(* Logix 5000 AddOnInstructionDefinition export HI1734_Faceplate_IT_AOI; software revision 30.00; part 2 of 2 *)
(* tags used below, declared in another part *)
   Inp_hi1734 : HI:1734_WS:I:0;
   Out_hi1734 : HI:1734_WS:O:0;
   IT_Status : DINT;   // Integrated Technician status indication
   pm_49C8 : REAL;   // WAVERSAVER VAR ref 1
   pm_49C4 : REAL;   // WAVERSAVER VAR ch 4
   pm_49C5 : REAL;   // WAVERSAVER VAR ch 5
   pm_49C6 : REAL;   // WAVERSAVER VAR ch 6
   pm_49C7 : REAL;   // WAVERSAVER VAR ch 7
   pm_49C9 : REAL;   // WAVERSAVER VAR ref 2
   pm_49D0 : DINT;   // RAW VAR results ch 0
   pm_49D1 : DINT;   // RAW VAR results ch 1
   pm_49D2 : DINT;   // RAW VAR results ch 2
   pm_49D3 : DINT;   // RAW VAR results ch 3
   pm_49D8 : DINT;   // RAW VAR results ref 1
   pm_49D4 : DINT;   // RAW VAR results ch 4
   pm_49D5 : DINT;   // RAW VAR results ch 5
   pm_49D6 : DINT;   // RAW VAR results ch 6
   pm_49D7 : DINT;   // RAW VAR results ch 7
   pm_49D9 : DINT;   // RAW VAR results ref 2
   pm_49E0 : DINT;   // WAVERSAVER VAR results ch 0
   pm_49E1 : DINT;   // WAVERSAVER VAR results ch 1
   pm_49E2 : DINT;   // WAVERSAVER VAR results ch 2
   pm_49E3 : DINT;   // WAVERSAVER VAR results ch 3
   pm_49E8 : DINT;   // WAVERSAVER VAR results ref 1
   pm_49E4 : DINT;   // WAVERSAVER VAR results ch 4
   pm_49E5 : DINT;   // WAVERSAVER VAR results ch 5
   pm_49E6 : DINT;   // WAVERSAVER VAR results ch 6
   pm_49E7 : DINT;   // WAVERSAVER VAR results ch 7
   pm_49E9 : DINT;   // WAVERSAVER VAR results ref 2
   rd_rtz : INT;   // return to zero status
   pm_49F0 : DINT;   // RTZ ch 0
   pm_49F1 : DINT;   // RTZ ch 1
   pm_49F2 : DINT;   // RTZ ch 2
   pm_49F3 : DINT;   // RTZ ch 3
   pm_49F4 : DINT;   // RTZ ch 4
   pm_49F5 : DINT;   // RTZ ch 5
   pm_49F6 : DINT;   // RTZ ch 6
   pm_49F7 : DINT;   // RTZ ch 7
   pm_498C : DINT;   // RTZ combined
   IT_running_status : DINT;   // running/status indication
   rd_ws_var : INT;   // trigger to read WAVERSAVER variation
   rd_raw_rst : INT;   // trigger to read raw variation results
   rd_ws_rst : INT;   // trigger to read WAVERSAVER results
   start_timer116 : BOOL;   // process control bit
   delay116 : TIMER;   // delay to allow process to complete
   start_timer117 : BOOL;   // process control bit
   delay117 : TIMER;   // delay to allow process to complete
   start_timer118 : BOOL;   // process control bit
   start_timer119 : BOOL;   // process control bit
   delay118 : TIMER;   // delay to allow process to complete
   delay119 : TIMER;   // delay to allow process to complete
   start_timer120 : BOOL;   // process control bit
   delay120 : TIMER;   // delay to allow process to complete
   start_timer121 : BOOL;   // process control bit
   delay121 : TIMER;   // delay to allow process to complete
   start_timer122 : BOOL;   // process control bit
   delay122 : TIMER;   // delay to allow process to complete
   start_timer123 : BOOL;   // process control bit
   delay123 : TIMER;   // delay to allow process to complete
   start_timer124 : BOOL;   // process control bit
   delay124 : TIMER;   // delay to allow process to complete
   start_timer125 : BOOL;   // process control bit
   delay125 : TIMER;   // delay to allow process to complete
   start_timer126 : BOOL;   // process control bit
   delay126 : TIMER;   // delay to allow process to complete
   start_timer127 : BOOL;   // process control bit
   delay127 : TIMER;   // delay to allow process to complete
   start_timer128 : BOOL;   // process control bit
   delay128 : TIMER;   // delay to allow process to complete
   start_timer129 : BOOL;   // process control bit
   delay129 : TIMER;   // delay to allow process to complete
   start_timer130 : BOOL;   // process control bit
   delay130 : TIMER;   // delay to allow process to complete
   start_timer131 : BOOL;   // process control bit
   delay131 : TIMER;   // delay to allow process to complete
   start_timer132 : BOOL;   // process control bit
   delay132 : TIMER;   // delay to allow process to complete
   start_timer133 : BOOL;   // process control bit
   delay133 : TIMER;   // delay to allow process to complete
   clear_status : BOOL;   // process control bit
   delay138 : TIMER;   // delay to allow process to complete
   rd_jbox_2_too : BOOL;   // Process control bit
(* HI1734_Faceplate_IT_AOI, continued *)

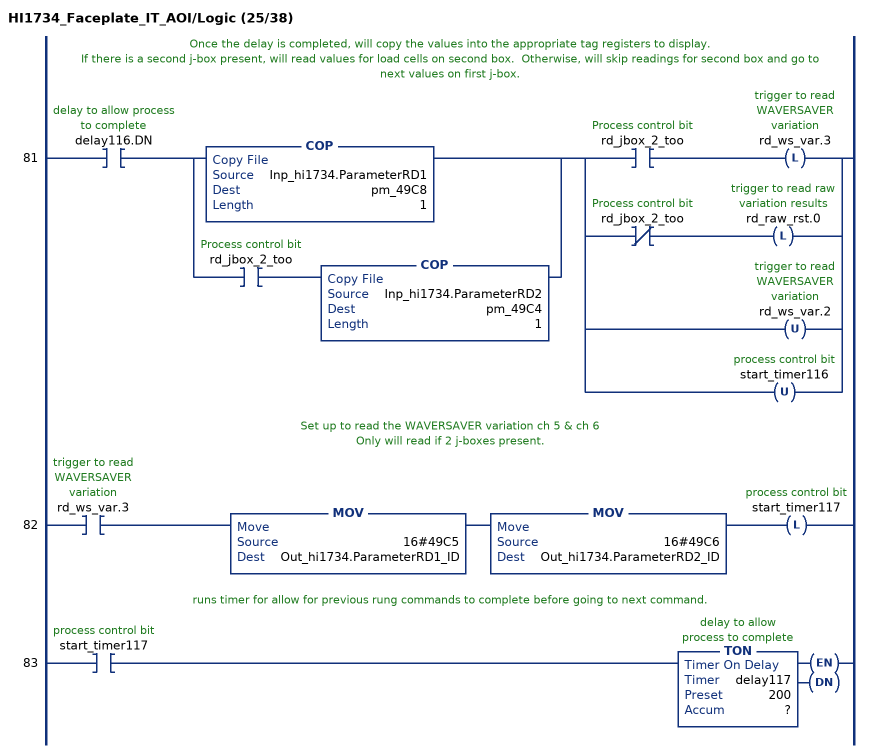
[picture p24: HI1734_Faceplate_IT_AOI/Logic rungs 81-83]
   // Once the delay is completed, will copy the values into the appropriate tag registers to display.
   // If there is a second j-box present, will read values for load cells on second box.  Otherwise, will skip readings for second box and go to next values on first j-box.
   81: XIC(delay116.DN)[COP(Inp_hi1734.ParameterRD1,pm_49C8,1) ,XIC(rd_jbox_2_too) COP(Inp_hi1734.ParameterRD2,pm_49C4,1) ][XIC(rd_jbox_2_too) OTL(rd_ws_var.3) ,XIO(rd_jbox_2_too) OTL(rd_raw_rst.0) ,OTU(rd_ws_var.2) ,OTU(start_timer116) ];
   // Set up to read the WAVERSAVER variation ch 5 & ch 6
   // Only will read if 2 j-boxes present.
   82: XIC(rd_ws_var.3)MOV(16#49C5,Out_hi1734.ParameterRD1_ID)MOV(16#49C6,Out_hi1734.ParameterRD2_ID)OTL(start_timer117);
   // runs timer for allow for previous rung commands to complete before going to next command.
   83: XIC(start_timer117)TON(delay117,?,?);
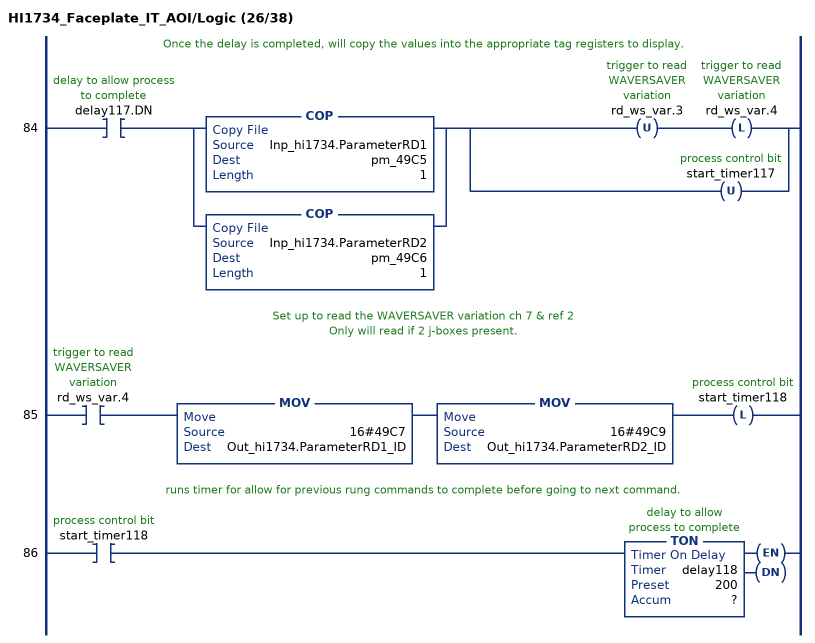
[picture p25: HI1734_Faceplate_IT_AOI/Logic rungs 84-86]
   // Once the delay is completed, will copy the values into the appropriate tag registers to display.
   84: XIC(delay117.DN)[COP(Inp_hi1734.ParameterRD1,pm_49C5,1) ,COP(Inp_hi1734.ParameterRD2,pm_49C6,1) ][OTU(rd_ws_var.3) OTL(rd_ws_var.4) ,OTU(start_timer117) ];
   // Set up to read the WAVERSAVER variation ch 7 & ref 2
   // Only will read if 2 j-boxes present.
   85: XIC(rd_ws_var.4)MOV(16#49C7,Out_hi1734.ParameterRD1_ID)MOV(16#49C9,Out_hi1734.ParameterRD2_ID)OTL(start_timer118);
   // runs timer for allow for previous rung commands to complete before going to next command.
   86: XIC(start_timer118)TON(delay118,?,?);
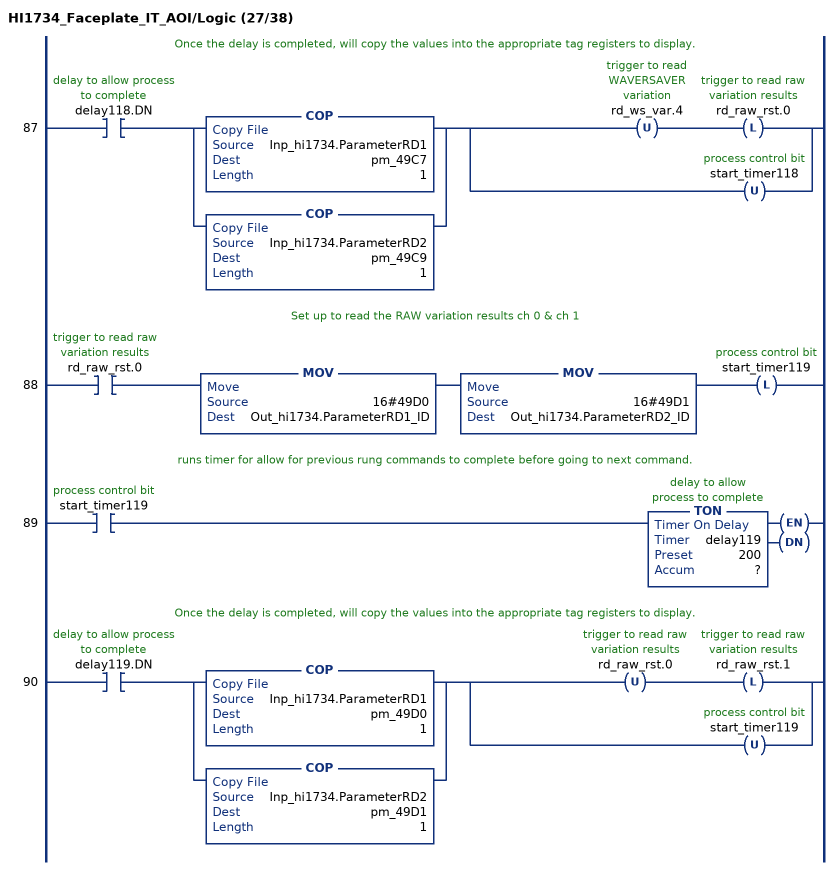
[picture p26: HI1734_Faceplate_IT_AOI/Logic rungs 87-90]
   // Once the delay is completed, will copy the values into the appropriate tag registers to display.
   87: XIC(delay118.DN)[COP(Inp_hi1734.ParameterRD1,pm_49C7,1) ,COP(Inp_hi1734.ParameterRD2,pm_49C9,1) ][OTU(rd_ws_var.4) OTL(rd_raw_rst.0) ,OTU(start_timer118) ];
   // Set up to read the RAW variation results ch 0 & ch 1
   88: XIC(rd_raw_rst.0)MOV(16#49D0,Out_hi1734.ParameterRD1_ID)MOV(16#49D1,Out_hi1734.ParameterRD2_ID)OTL(start_timer119);
   // runs timer for allow for previous rung commands to complete before going to next command.
   89: XIC(start_timer119)TON(delay119,?,?);
   // Once the delay is completed, will copy the values into the appropriate tag registers to display.
   90: XIC(delay119.DN)[COP(Inp_hi1734.ParameterRD1,pm_49D0,1) ,COP(Inp_hi1734.ParameterRD2,pm_49D1,1) ][OTU(rd_raw_rst.0) OTL(rd_raw_rst.1) ,OTU(start_timer119) ];
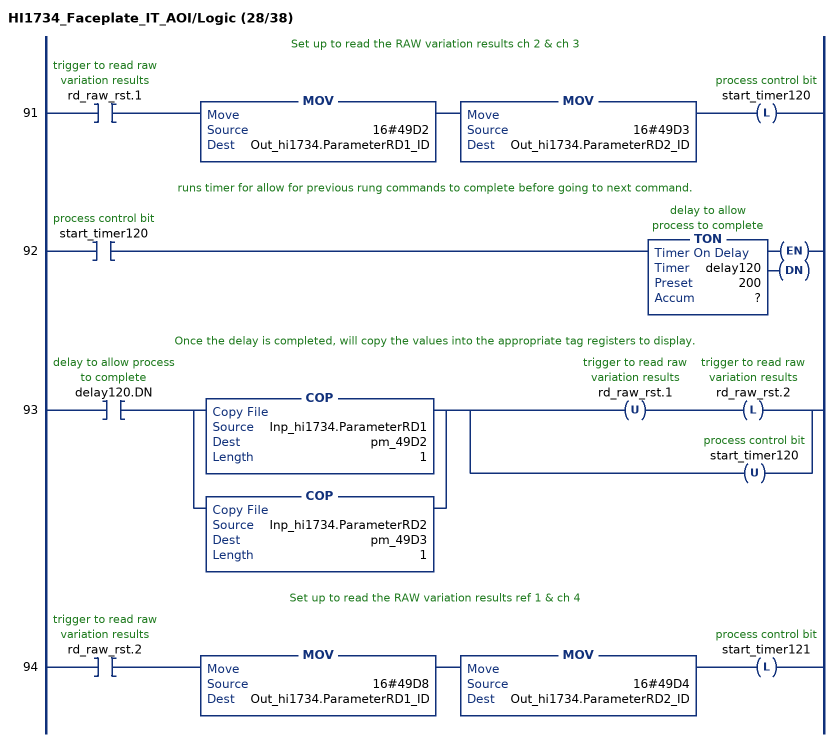
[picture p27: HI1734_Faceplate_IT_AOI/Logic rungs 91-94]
   // Set up to read the RAW variation results ch 2 & ch 3
   91: XIC(rd_raw_rst.1)MOV(16#49D2,Out_hi1734.ParameterRD1_ID)MOV(16#49D3,Out_hi1734.ParameterRD2_ID)OTL(start_timer120);
   // runs timer for allow for previous rung commands to complete before going to next command.
   92: XIC(start_timer120)TON(delay120,?,?);
   // Once the delay is completed, will copy the values into the appropriate tag registers to display.
   93: XIC(delay120.DN)[COP(Inp_hi1734.ParameterRD1,pm_49D2,1) ,COP(Inp_hi1734.ParameterRD2,pm_49D3,1) ][OTU(rd_raw_rst.1) OTL(rd_raw_rst.2) ,OTU(start_timer120) ];
   // Set up to read the RAW variation results ref 1 & ch 4
   94: XIC(rd_raw_rst.2)MOV(16#49D8,Out_hi1734.ParameterRD1_ID)MOV(16#49D4,Out_hi1734.ParameterRD2_ID)OTL(start_timer121);
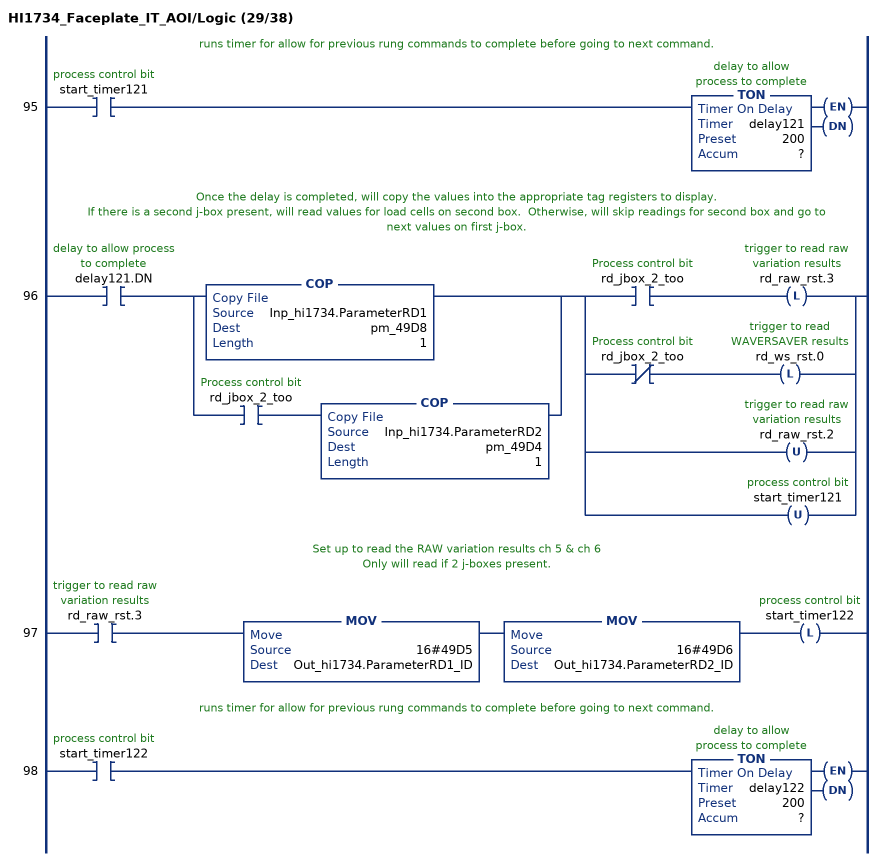
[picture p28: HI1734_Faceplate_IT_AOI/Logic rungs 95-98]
   // runs timer for allow for previous rung commands to complete before going to next command.
   95: XIC(start_timer121)TON(delay121,?,?);
   // Once the delay is completed, will copy the values into the appropriate tag registers to display.
   // If there is a second j-box present, will read values for load cells on second box.  Otherwise, will skip readings for second box and go to next values on first j-box.
   96: XIC(delay121.DN)[COP(Inp_hi1734.ParameterRD1,pm_49D8,1) ,XIC(rd_jbox_2_too) COP(Inp_hi1734.ParameterRD2,pm_49D4,1) ][XIC(rd_jbox_2_too) OTL(rd_raw_rst.3) ,XIO(rd_jbox_2_too) OTL(rd_ws_rst.0) ,OTU(rd_raw_rst.2) ,OTU(start_timer121) ];
   // Set up to read the RAW variation results ch 5 & ch 6
   // Only will read if 2 j-boxes present.
   97: XIC(rd_raw_rst.3)MOV(16#49D5,Out_hi1734.ParameterRD1_ID)MOV(16#49D6,Out_hi1734.ParameterRD2_ID)OTL(start_timer122);
   // runs timer for allow for previous rung commands to complete before going to next command.
   98: XIC(start_timer122)TON(delay122,?,?);
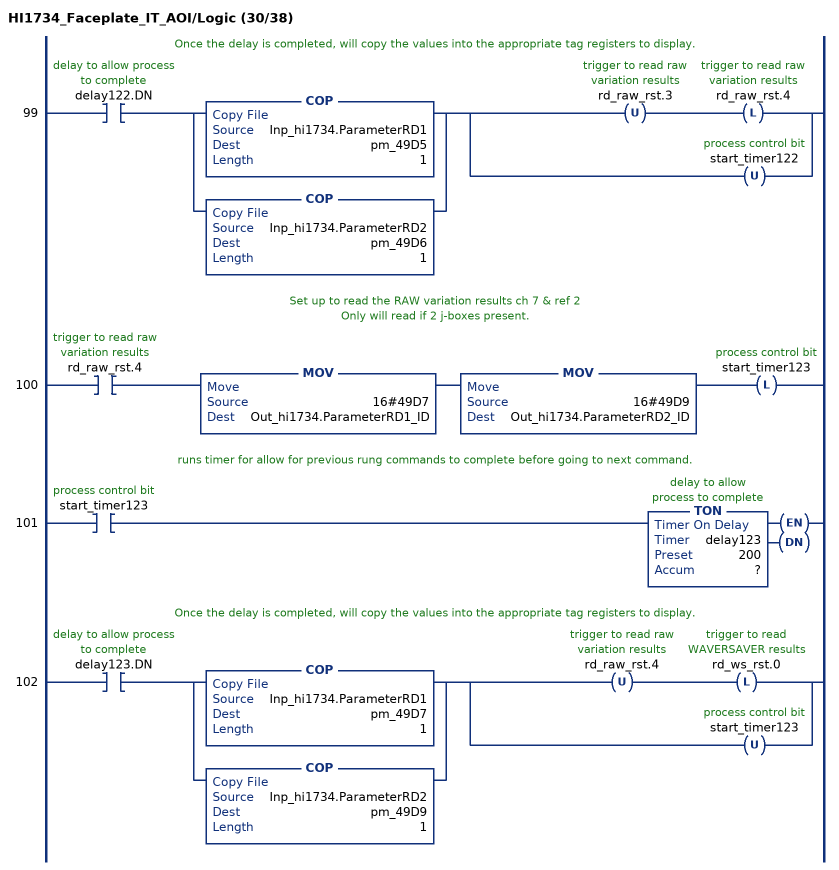
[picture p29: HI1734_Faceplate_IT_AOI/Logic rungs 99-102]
   // Once the delay is completed, will copy the values into the appropriate tag registers to display.
   99: XIC(delay122.DN)[COP(Inp_hi1734.ParameterRD1,pm_49D5,1) ,COP(Inp_hi1734.ParameterRD2,pm_49D6,1) ][OTU(rd_raw_rst.3) OTL(rd_raw_rst.4) ,OTU(start_timer122) ];
   // Set up to read the RAW variation results ch 7 & ref 2
   // Only will read if 2 j-boxes present.
   100: XIC(rd_raw_rst.4)MOV(16#49D7,Out_hi1734.ParameterRD1_ID)MOV(16#49D9,Out_hi1734.ParameterRD2_ID)OTL(start_timer123);
   // runs timer for allow for previous rung commands to complete before going to next command.
   101: XIC(start_timer123)TON(delay123,?,?);
   // Once the delay is completed, will copy the values into the appropriate tag registers to display.
   102: XIC(delay123.DN)[COP(Inp_hi1734.ParameterRD1,pm_49D7,1) ,COP(Inp_hi1734.ParameterRD2,pm_49D9,1) ][OTU(rd_raw_rst.4) OTL(rd_ws_rst.0) ,OTU(start_timer123) ];
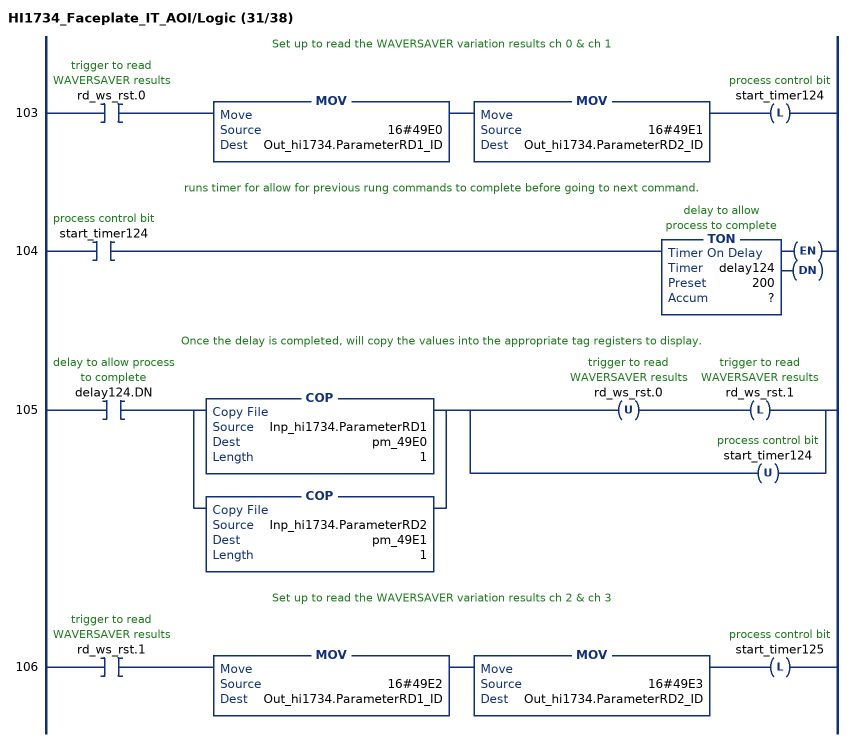
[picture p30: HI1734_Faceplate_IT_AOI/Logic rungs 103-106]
   // Set up to read the WAVERSAVER variation results ch 0 & ch 1
   103: XIC(rd_ws_rst.0)MOV(16#49E0,Out_hi1734.ParameterRD1_ID)MOV(16#49E1,Out_hi1734.ParameterRD2_ID)OTL(start_timer124);
   // runs timer for allow for previous rung commands to complete before going to next command.
   104: XIC(start_timer124)TON(delay124,?,?);
   // Once the delay is completed, will copy the values into the appropriate tag registers to display.
   105: XIC(delay124.DN)[COP(Inp_hi1734.ParameterRD1,pm_49E0,1) ,COP(Inp_hi1734.ParameterRD2,pm_49E1,1) ][OTU(rd_ws_rst.0) OTL(rd_ws_rst.1) ,OTU(start_timer124) ];
   // Set up to read the WAVERSAVER variation results ch 2 & ch 3
   106: XIC(rd_ws_rst.1)MOV(16#49E2,Out_hi1734.ParameterRD1_ID)MOV(16#49E3,Out_hi1734.ParameterRD2_ID)OTL(start_timer125);
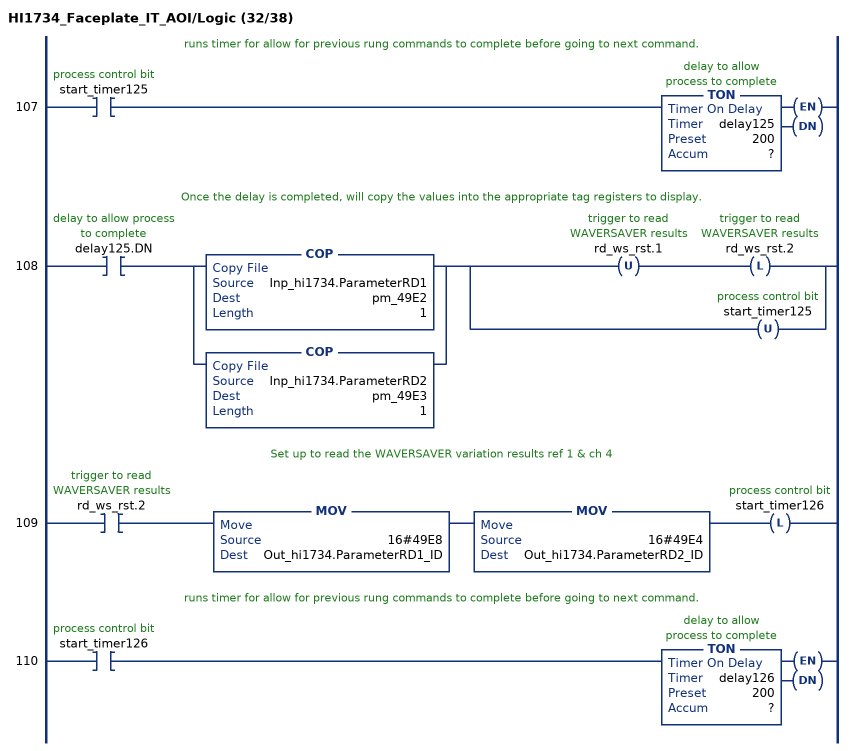
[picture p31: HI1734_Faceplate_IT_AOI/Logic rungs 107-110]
   // runs timer for allow for previous rung commands to complete before going to next command.
   107: XIC(start_timer125)TON(delay125,?,?);
   // Once the delay is completed, will copy the values into the appropriate tag registers to display.
   108: XIC(delay125.DN)[COP(Inp_hi1734.ParameterRD1,pm_49E2,1) ,COP(Inp_hi1734.ParameterRD2,pm_49E3,1) ][OTU(rd_ws_rst.1) OTL(rd_ws_rst.2) ,OTU(start_timer125) ];
   // Set up to read the WAVERSAVER variation results ref 1 & ch 4
   109: XIC(rd_ws_rst.2)MOV(16#49E8,Out_hi1734.ParameterRD1_ID)MOV(16#49E4,Out_hi1734.ParameterRD2_ID)OTL(start_timer126);
   // runs timer for allow for previous rung commands to complete before going to next command.
   110: XIC(start_timer126)TON(delay126,?,?);
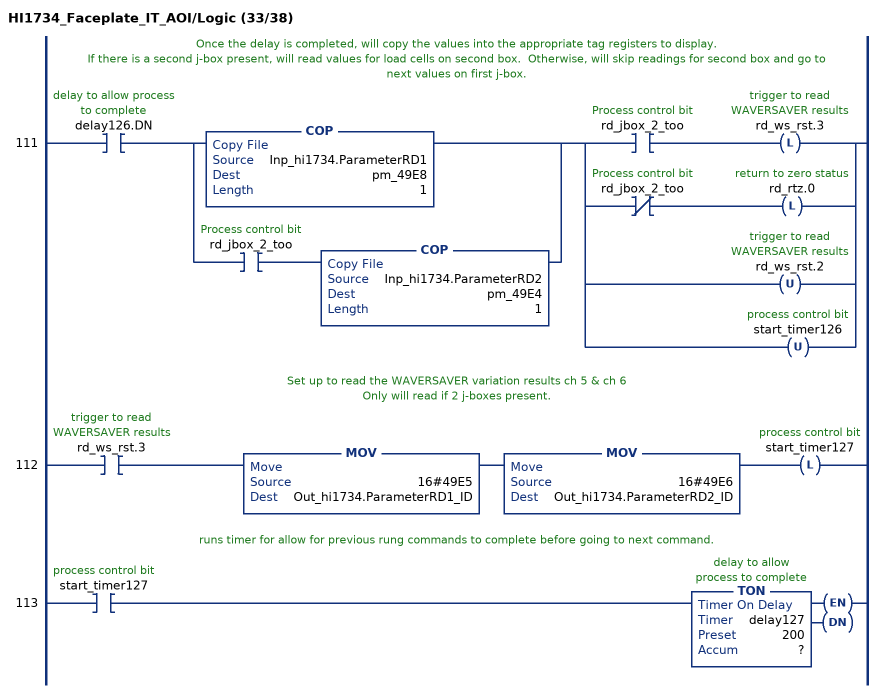
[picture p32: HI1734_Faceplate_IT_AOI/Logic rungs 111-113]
   // Once the delay is completed, will copy the values into the appropriate tag registers to display.
   // If there is a second j-box present, will read values for load cells on second box.  Otherwise, will skip readings for second box and go to next values on first j-box.
   111: XIC(delay126.DN)[COP(Inp_hi1734.ParameterRD1,pm_49E8,1) ,XIC(rd_jbox_2_too) COP(Inp_hi1734.ParameterRD2,pm_49E4,1) ][XIC(rd_jbox_2_too) OTL(rd_ws_rst.3) ,XIO(rd_jbox_2_too) OTL(rd_rtz.0) ,OTU(rd_ws_rst.2) ,OTU(start_timer126) ];
   // Set up to read the WAVERSAVER variation results ch 5 & ch 6
   // Only will read if 2 j-boxes present.
   112: XIC(rd_ws_rst.3)MOV(16#49E5,Out_hi1734.ParameterRD1_ID)MOV(16#49E6,Out_hi1734.ParameterRD2_ID)OTL(start_timer127);
   // runs timer for allow for previous rung commands to complete before going to next command.
   113: XIC(start_timer127)TON(delay127,?,?);
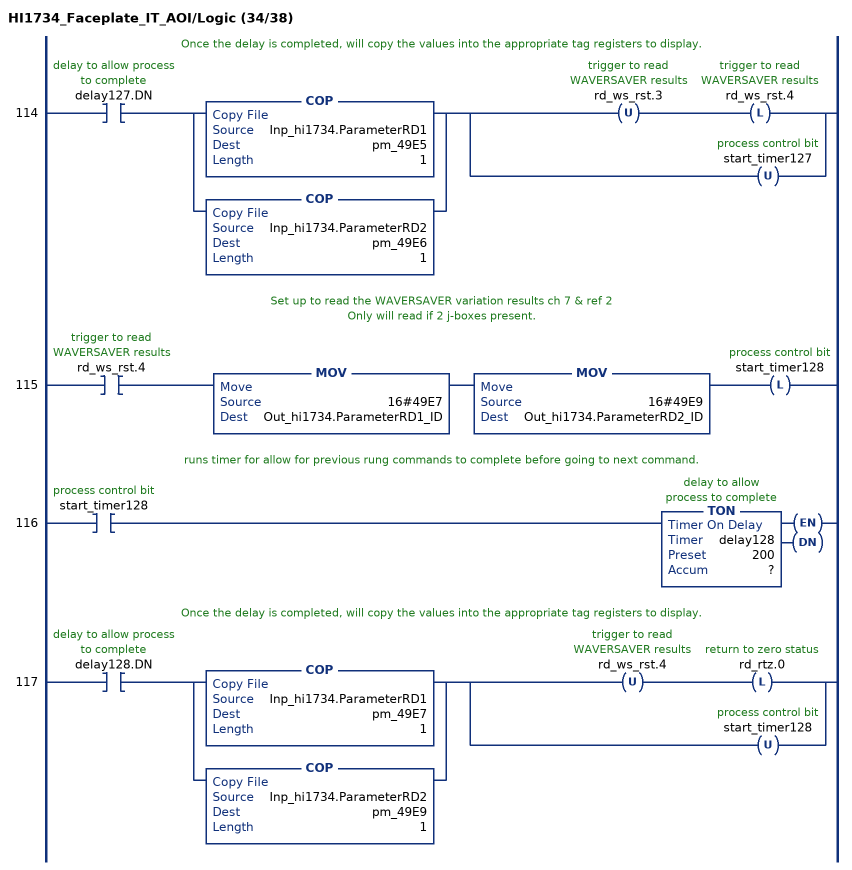
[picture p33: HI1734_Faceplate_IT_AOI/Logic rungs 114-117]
   // Once the delay is completed, will copy the values into the appropriate tag registers to display.
   114: XIC(delay127.DN)[COP(Inp_hi1734.ParameterRD1,pm_49E5,1) ,COP(Inp_hi1734.ParameterRD2,pm_49E6,1) ][OTU(rd_ws_rst.3) OTL(rd_ws_rst.4) ,OTU(start_timer127) ];
   // Set up to read the WAVERSAVER variation results ch 7 & ref 2
   //  Only will read if 2 j-boxes present.
   115: XIC(rd_ws_rst.4)MOV(16#49E7,Out_hi1734.ParameterRD1_ID)MOV(16#49E9,Out_hi1734.ParameterRD2_ID)OTL(start_timer128);
   // runs timer for allow for previous rung commands to complete before going to next command.
   116: XIC(start_timer128)TON(delay128,?,?);
   // Once the delay is completed, will copy the values into the appropriate tag registers to display.
   117: XIC(delay128.DN)[COP(Inp_hi1734.ParameterRD1,pm_49E7,1) ,COP(Inp_hi1734.ParameterRD2,pm_49E9,1) ][OTU(rd_ws_rst.4) OTL(rd_rtz.0) ,OTU(start_timer128) ];
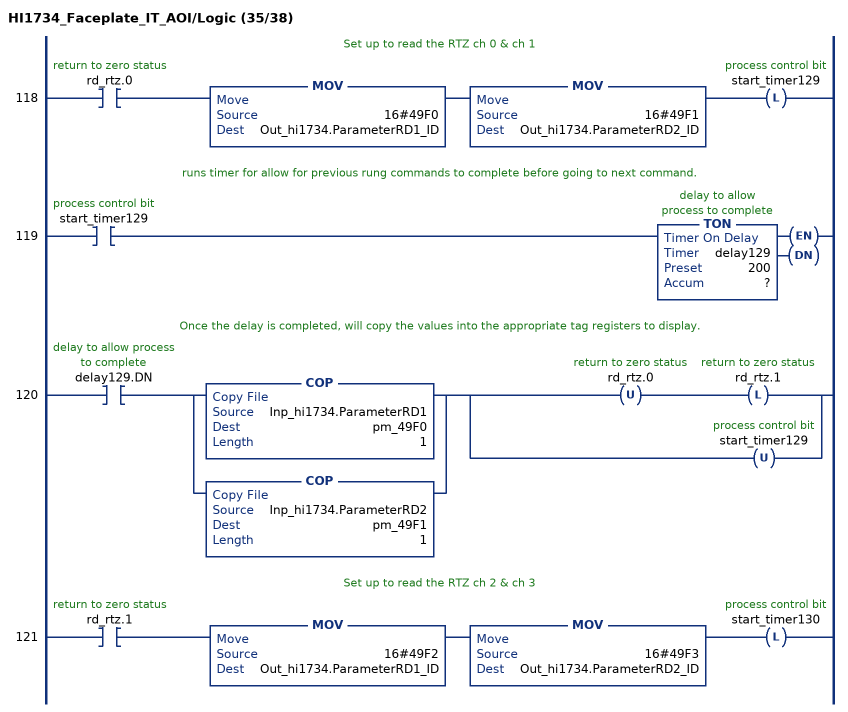
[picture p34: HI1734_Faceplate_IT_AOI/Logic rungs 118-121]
   // Set up to read the RTZ ch 0 & ch 1
   118: XIC(rd_rtz.0)MOV(16#49F0,Out_hi1734.ParameterRD1_ID)MOV(16#49F1,Out_hi1734.ParameterRD2_ID)OTL(start_timer129);
   // runs timer for allow for previous rung commands to complete before going to next command.
   119: XIC(start_timer129)TON(delay129,?,?);
   // Once the delay is completed, will copy the values into the appropriate tag registers to display.
   120: XIC(delay129.DN)[COP(Inp_hi1734.ParameterRD1,pm_49F0,1) ,COP(Inp_hi1734.ParameterRD2,pm_49F1,1) ][OTU(rd_rtz.0) OTL(rd_rtz.1) ,OTU(start_timer129) ];
   // Set up to read the RTZ ch 2 & ch 3
   121: XIC(rd_rtz.1)MOV(16#49F2,Out_hi1734.ParameterRD1_ID)MOV(16#49F3,Out_hi1734.ParameterRD2_ID)OTL(start_timer130);
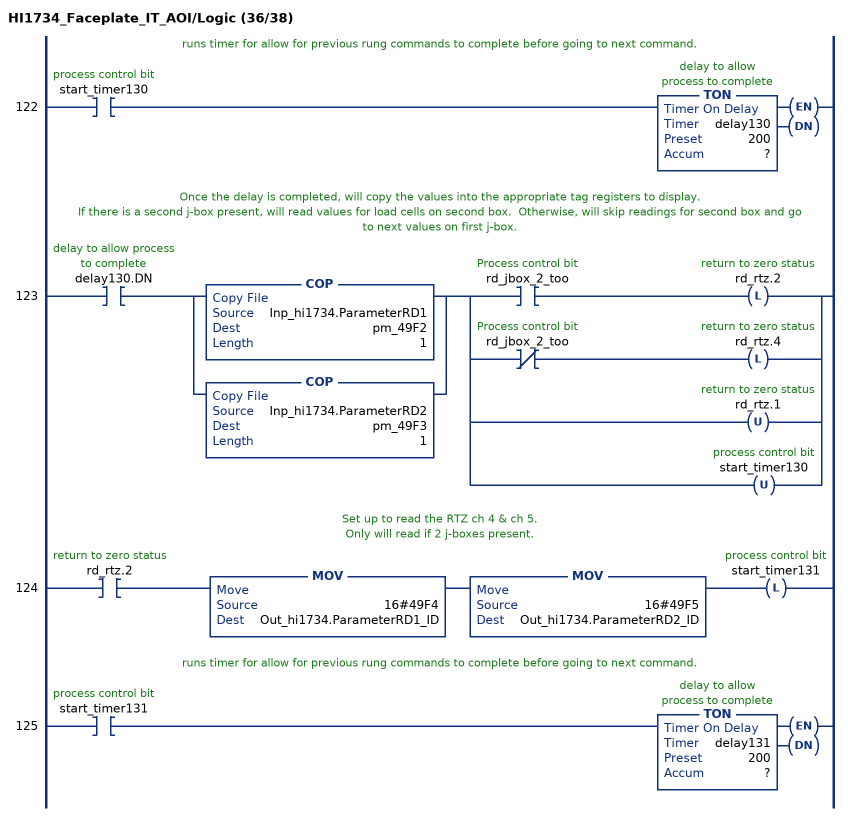
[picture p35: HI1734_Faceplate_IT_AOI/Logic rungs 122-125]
   // runs timer for allow for previous rung commands to complete before going to next command.
   122: XIC(start_timer130)TON(delay130,?,?);
   // Once the delay is completed, will copy the values into the appropriate tag registers to display.
   // If there is a second j-box present, will read values for load cells on second box.  Otherwise, will skip readings for second box and go to next values on first j-box.
   123: XIC(delay130.DN)[COP(Inp_hi1734.ParameterRD1,pm_49F2,1) ,COP(Inp_hi1734.ParameterRD2,pm_49F3,1) ][XIC(rd_jbox_2_too) OTL(rd_rtz.2) ,XIO(rd_jbox_2_too) OTL(rd_rtz.4) ,OTU(rd_rtz.1) ,OTU(start_timer130) ];
   // Set up to read the RTZ ch 4 & ch 5.
   // Only will read if 2 j-boxes present.
   124: XIC(rd_rtz.2)MOV(16#49F4,Out_hi1734.ParameterRD1_ID)MOV(16#49F5,Out_hi1734.ParameterRD2_ID)OTL(start_timer131);
   // runs timer for allow for previous rung commands to complete before going to next command.
   125: XIC(start_timer131)TON(delay131,?,?);
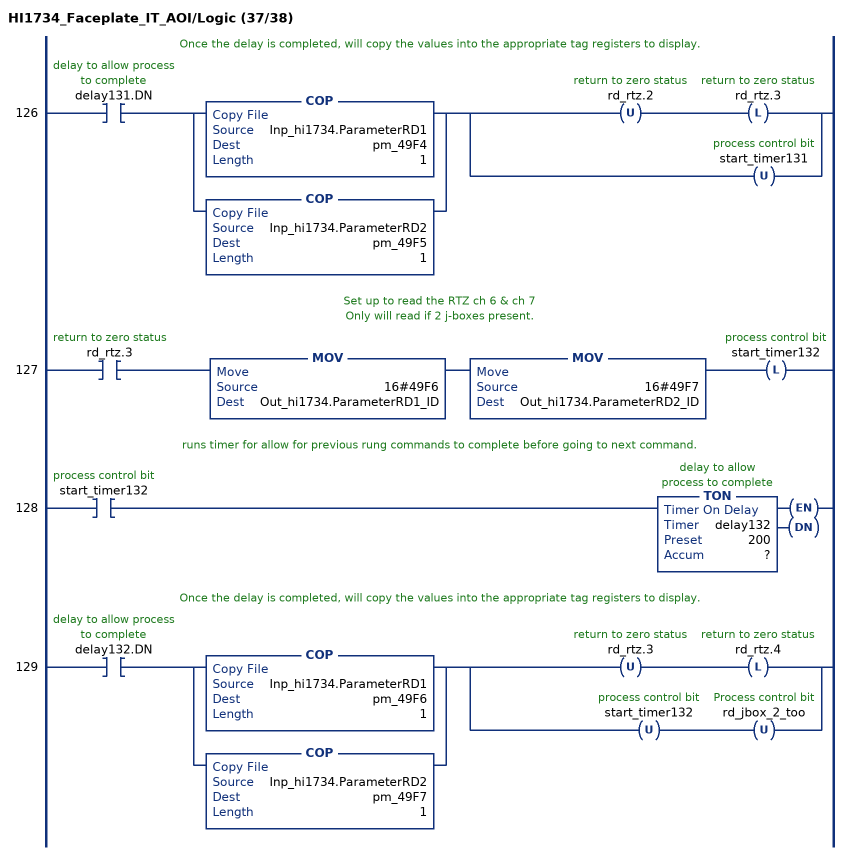
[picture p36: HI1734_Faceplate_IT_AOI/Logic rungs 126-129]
   // Once the delay is completed, will copy the values into the appropriate tag registers to display.
   126: XIC(delay131.DN)[COP(Inp_hi1734.ParameterRD1,pm_49F4,1) ,COP(Inp_hi1734.ParameterRD2,pm_49F5,1) ][OTU(rd_rtz.2) OTL(rd_rtz.3) ,OTU(start_timer131) ];
   // Set up to read the RTZ ch 6 & ch 7
   // Only will read if 2 j-boxes present.
   127: XIC(rd_rtz.3)MOV(16#49F6,Out_hi1734.ParameterRD1_ID)MOV(16#49F7,Out_hi1734.ParameterRD2_ID)OTL(start_timer132);
   // runs timer for allow for previous rung commands to complete before going to next command.
   128: XIC(start_timer132)TON(delay132,?,?);
   // Once the delay is completed, will copy the values into the appropriate tag registers to display.
   129: XIC(delay132.DN)[COP(Inp_hi1734.ParameterRD1,pm_49F6,1) ,COP(Inp_hi1734.ParameterRD2,pm_49F7,1) ][OTU(rd_rtz.3) OTL(rd_rtz.4) ,OTU(start_timer132) OTU(rd_jbox_2_too) ];
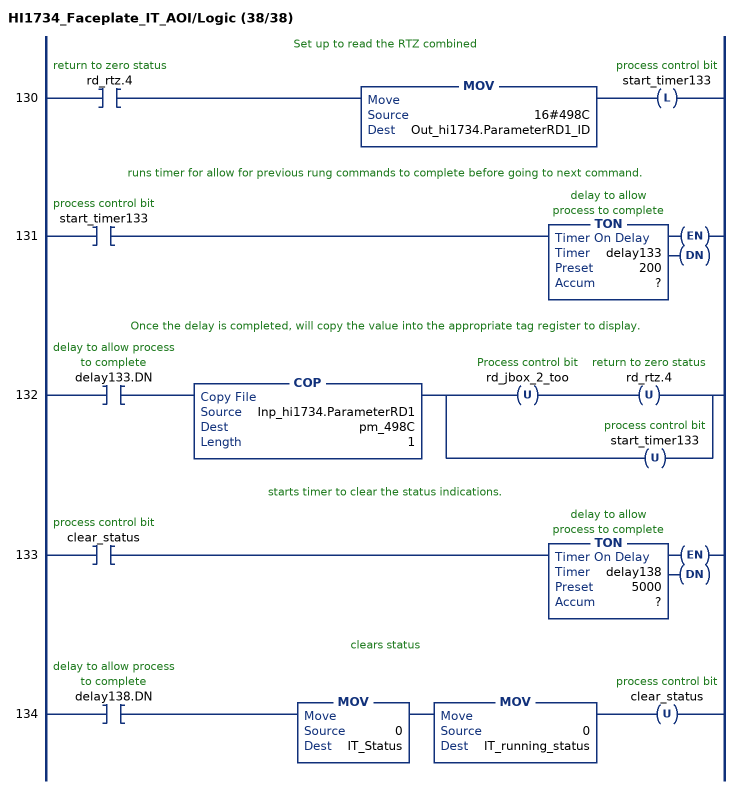
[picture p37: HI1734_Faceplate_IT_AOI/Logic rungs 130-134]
   // Set up to read the RTZ combined
   130: XIC(rd_rtz.4)MOV(16#498C,Out_hi1734.ParameterRD1_ID)OTL(start_timer133);
   // runs timer for allow for previous rung commands to complete before going to next command.
   131: XIC(start_timer133)TON(delay133,?,?);
   // Once the delay is completed, will copy the value into the appropriate tag register to display.
   132: XIC(delay133.DN)COP(Inp_hi1734.ParameterRD1,pm_498C,1)[OTU(rd_jbox_2_too) OTU(rd_rtz.4) ,OTU(start_timer133) ];
   // starts timer to clear the status indications.
   133: XIC(clear_status)TON(delay138,?,?);
   // clears status
   134: XIC(delay138.DN)MOV(0,IT_Status)MOV(0,IT_running_status)OTU(clear_status);
END_ROUTINE
END_ADD_ON_INSTRUCTION
